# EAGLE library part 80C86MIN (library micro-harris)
MICROCONTROLLER/MEMORY DEVICE
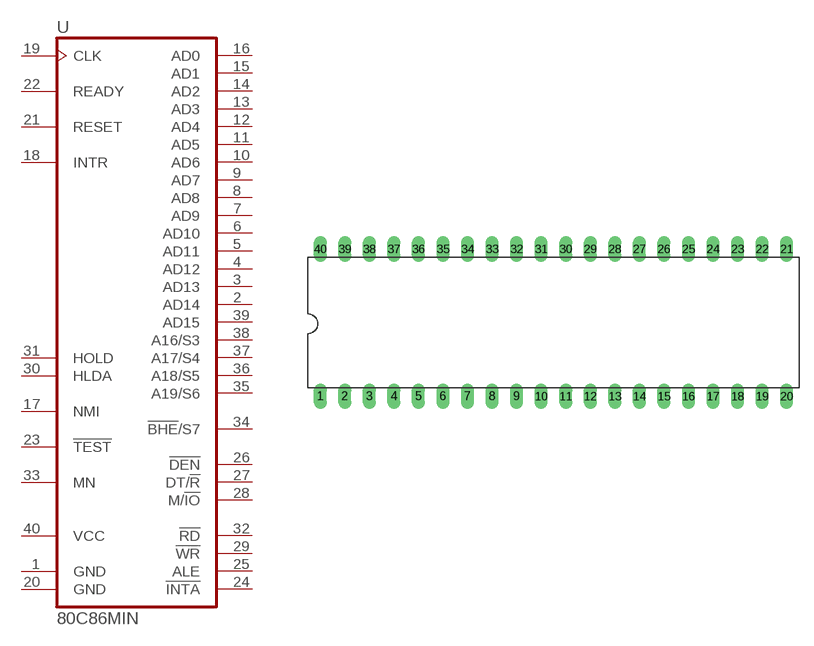
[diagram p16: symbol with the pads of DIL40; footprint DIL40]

Designator prefix U

## 80C86MIN (MPN: CP80C86-2; OC_FARNELL: unknown; OC_NEWARK: 16F4891)  [DIL40]
1  GND  pwr
2  AD14
3  AD13
4  AD12
5  AD11
6  AD10
7  AD9
8  AD8
9  AD7
10  AD6
11  AD5
12  AD4
13  AD3
14  AD2
15  AD1
16  AD0
17  NMI  in
18  INTR  in
19  CLK  in
20  GND  pwr
21  RESET  in
22  READY  in
23  !TEST  in
24  !INTA  out
25  ALE  out
26  !DEN  out
27  DT/!R  out
28  M/!IO  out
29  !WR  out
30  HLDA  out
31  HOLD  in
32  !RD  out
33  MN  in
34  !BHE!/S7  out
35  A19/S6  out
36  A18/S5  out
37  A17/S4  out
38  A16/S3  out
39  AD15
40  VCC  pwr

## Footprint DIL40 (pad centres in mm)
Dual In Line Package
drill 0.813 long: 1 -24.13,-7.62; 2 -21.59,-7.62; 3 -19.05,-7.62; 4 -16.51,-7.62; 5 -13.97,-7.62; 6 -11.43,-7.62; 7 -8.89,-7.62; 8 -6.35,-7.62; 9 -3.81,-7.62; 10 -1.27,-7.62; 11 1.27,-7.62; 12 3.81,-7.62; 13 6.35,-7.62; 14 8.89,-7.62; 15 11.43,-7.62; 16 13.97,-7.62; 17 16.51,-7.62; 18 19.05,-7.62; 19 21.59,-7.62; 20 24.13,-7.62; 21 24.13,7.62; 22 21.59,7.62; 23 19.05,7.62; 24 16.51,7.62; 25 13.97,7.62; 26 11.43,7.62; 27 8.89,7.62; 28 6.35,7.62; 29 3.81,7.62; 30 1.27,7.62; 31 -1.27,7.62; 32 -3.81,7.62; 33 -6.35,7.62; 34 -8.89,7.62; 35 -11.43,7.62; 36 -13.97,7.62; 37 -16.51,7.62; 38 -19.05,7.62; 39 -21.59,7.62; 40 -24.13,7.62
